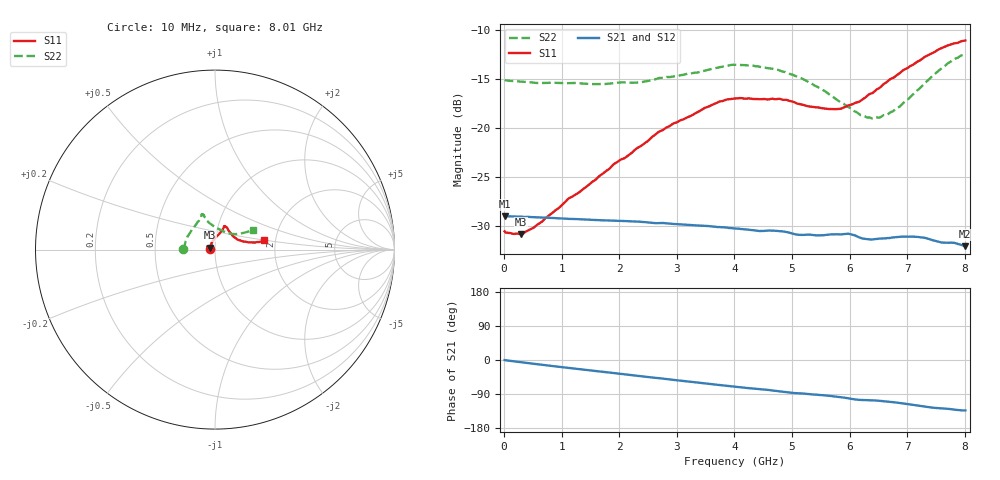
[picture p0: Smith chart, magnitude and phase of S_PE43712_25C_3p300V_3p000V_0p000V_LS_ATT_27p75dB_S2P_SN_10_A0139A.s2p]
! DEVICE ID: PE43712
! File Path: z:\PE43713\PE43713_CHAR_NOM_04292014\AMB\3p300\LS_ATT_27p75dB\PE43713_AMB_3p300V_3p000V_0p000V_LS_ATT_27p75dB_S2P_SN_10_A0139A.s2p
! Serial: 10
! Lot: A0139A
! Temp: 25C
! VDD: 3.300
! VSS: 0.000
! Control_Hi: 3.000
! Control_Lo: 0.000
! Attenuation Step: 27.75dB
! Port 1: RF1
! Port 2: RF2
! ThroughPath:1-2
! IDD: 0.0001455229
! ISS: -9.96e-008
#  Hz  S  RI  R  50
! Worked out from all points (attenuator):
!   801 points, 10 MHz to 8.01 GHz, reference 50 ohm
!   highest |S21| = -29.01 dB at 10 MHz (marker M1); lowest = -32.1 dB at 8 GHz (marker M2)
!   lowest |S11| = -30.8 dB at 290 MHz (marker M3), VSWR 1.06, Z = 47.4 + j1.03 ohm
!   |S11| at or under -10 dB: start of sweep to end of sweep
!   |S22| runs from -19.1 to -12.5 dB; largest |S21 - S12| = 0.00014
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1e7  -0.0296 0.0008  0.0354 -0.000166  0.0355 -0.000163  -0.1756 0.00115
2.9e8  -0.0265 0.0109  0.0351 -0.00351  0.0351 -0.00351  -0.1714 0.0184
6.4e8  -0.0235 0.0231  0.0341 -0.00741  0.0341 -0.00742  -0.1653 0.0384
1.12e9  -0.0179 0.0397  0.0321 -0.0122  0.0321 -0.0123  -0.1566 0.0651
1.35e9  -0.0133 0.0463  0.031 -0.0144  0.031 -0.0144  -0.1507 0.076
2.3e9  0.0135 0.0774  0.0249 -0.022  0.0249 -0.022  -0.1163 0.1247
2.68e9  0.0267 0.0915  0.0219 -0.0242  0.0219 -0.0242  -0.1002 0.1491
3.5e9  0.0458 0.1187  0.0149 -0.0279  0.0149 -0.0279  -0.0769 0.1809
3.74e9  0.0496 0.1272  0.0127 -0.0285  0.0127 -0.0285  -0.0747 0.1904
4.01e9  0.0534 0.131  0.0103 -0.0289  0.0103 -0.0289  -0.074 0.197
4.76e9  0.0638 0.1257  0.00396 -0.0295  0.00401 -0.0295  -0.0605 0.1885
5.35e9  0.0803 0.0999  -0.00036 -0.0285  -0.000375 -0.0284  -0.0459 0.1616
5.82e9  0.1013 0.0734  -0.00393 -0.0283  -0.0039 -0.0284  -0.015 0.1358
6e9  0.1136 0.0653  -0.00589 -0.0281  -0.00583 -0.0281  0.000661 0.1271
6.2e9  0.1268 0.0552  -0.00729 -0.0264  -0.00726 -0.0264  0.0214 0.1141
6.41e9  0.1434 0.0496  -0.00769 -0.0259  -0.00763 -0.0258  0.0445 0.1022
6.68e9  0.1699 0.0436  -0.00937 -0.0257  -0.00933 -0.0257  0.0761 0.0909
7.16e9  0.2129 0.0397  -0.0137 -0.0242  -0.0137 -0.0241  0.1271 0.0877
7.55e9  0.2484 0.0433  -0.0159 -0.0209  -0.0158 -0.0208  0.1714 0.0966
7.81e9  0.266 0.0481  -0.0169 -0.0197  -0.0168 -0.0196  0.1973 0.1059
8e9  0.2746 0.0515  -0.017 -0.0182  -0.0169 -0.0182  0.2092 0.1096
8.01e9  0.2751 0.0521  -0.017 -0.0182  -0.017 -0.0182  0.2099 0.1096
